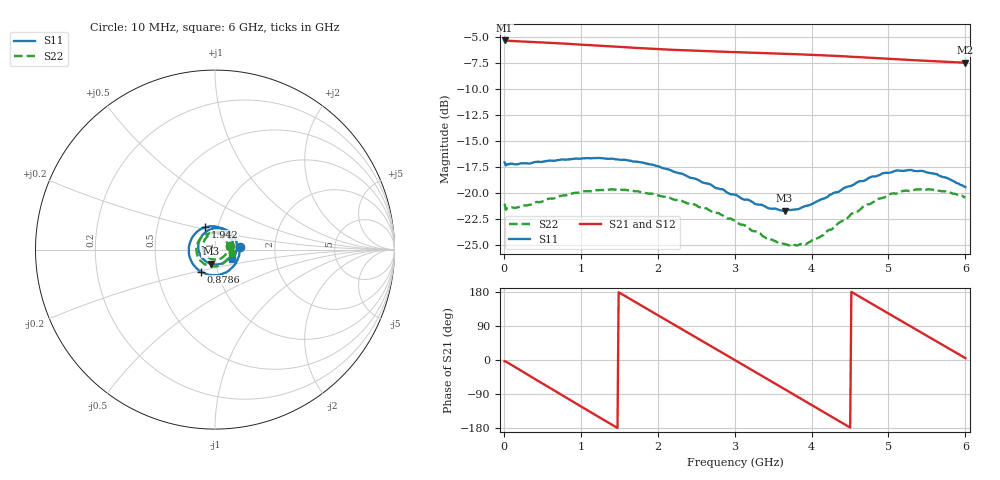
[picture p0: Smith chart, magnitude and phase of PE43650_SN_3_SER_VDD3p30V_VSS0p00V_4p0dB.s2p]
!Keysight Technologies,N5245B,MY57181451,A.13.50.07
!Date: Tuesday, May 07, 2019 07:59:52
!Correction: S11(Full 2 Port(1,2))
!S21(Full 2 Port(1,2))
!S12(Full 2 Port(1,2))
!S22(Full 2 Port(1,2))
!S2P File: Measurements: S11, S21, S12, S22:
# Hz S  dB  R 50
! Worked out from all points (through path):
!   401 points, 10 MHz to 6 GHz, reference 50 ohm
!   highest |S21| = -5.30 dB at 10 MHz (marker M1); lowest = -7.4 dB at 6 GHz (marker M2)
!   group delay of S21, straight-line fit = 330 ps
!   lowest |S11| = -21.7 dB at 3.649 GHz (marker M3), VSWR 1.18, Z = 47.1 - j7.43 ohm
!   |S11| at or under -10 dB: start of sweep to end of sweep
!   |S22| runs from -25.2 to -19.7 dB; largest |S21 - S12| = 0.004
!   S11 on the Smith chart (normalised r, x): 10 MHz: 1.32, +0.04; 878.5 MHz: 0.83, -0.21; 1.942 GHz: 0.87, +0.22; 6 GHz: 1.20, -0.13
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1e7  -17.07 6.4  -5.30 -3.3  -5.34 -3.3  -21.06 14.0
2.34625e8  -17.15 -34.5  -5.40 -29.4  -5.45 -29.4  -21.26 -35.1
4.892e8  -17.02 -70.3  -5.49 -60.5  -5.54 -60.4  -20.87 -71.7
8.7855e8  -16.74 -122.4  -5.64 -107.6  -5.69 -107.6  -20.08 -122.8
1.013325e9  -16.69 -139.4  -5.71 -123.8  -5.75 -123.8  -19.90 -139.1
1.252925e9  -16.65 -168.4  -5.81 -152.6  -5.87 -152.6  -19.73 -166.1
1.47755e9  -16.78 165.2  -5.90 -179.4  -5.97 -179.4  -19.72 169.5
1.941775e9  -17.30 113.1  -6.10 125.4  -6.16 125.4  -20.12 122.6
2.01665e9  -17.47 105.0  -6.13 116.5  -6.18 116.5  -20.27 115.4
2.4659e9  -18.60 54.5  -6.29 63.4  -6.34 63.4  -21.10 71.1
2.750425e9  -19.54 21.6  -6.37 29.7  -6.42 29.8  -21.93 41.2
3.005e9  -20.18 -11.0  -6.42 -0.4  -6.48 -0.3  -22.71 12.3
3.3045e9  -21.14 -53.3  -6.50 -36.0  -6.55 -35.8  -23.87 -27.8
3.648925e9  -21.73 -106.9  -6.59 -76.8  -6.63 -76.8  -24.94 -81.7
4.008325e9  -21.08 -164.2  -6.69 -119.5  -6.73 -119.5  -24.58 -144.0
4.2629e9  -20.13 158.5  -6.77 -149.9  -6.82 -149.8  -23.53 175.6
4.5025e9  -19.37 126.2  -6.86 -178.4  -6.91 -178.2  -22.16 141.1
4.7421e9  -18.57 96.2  -6.96 153.2  -7.02 153.4  -21.10 112.0
5.01165e9  -18.07 65.7  -7.07 121.4  -7.12 121.5  -20.16 81.0
5.4609e9  -17.93 18.9  -7.25 68.4  -7.30 68.6  -19.74 36.1
5.745425e9  -18.54 -7.8  -7.36 34.9  -7.40 35.0  -19.86 10.6
6e9  -19.45 -29.8  -7.45 5.0  -7.49 5.0  -20.46 -10.1
